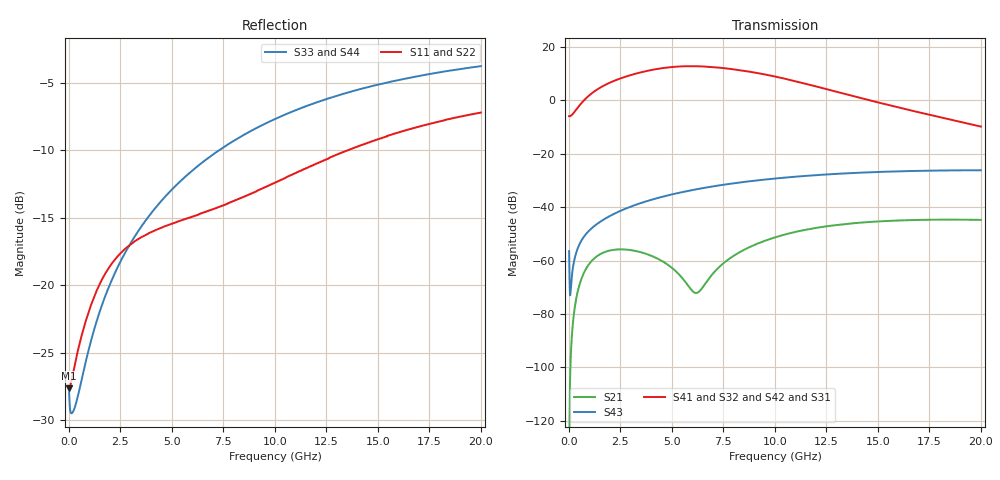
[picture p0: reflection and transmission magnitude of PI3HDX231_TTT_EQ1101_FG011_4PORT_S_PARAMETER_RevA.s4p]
! NPort=4 DATA=2000 NOISE=0 GROUPDELAY=0 COMPLEX_DATAFORMAT=POLAR
! NumOfBlock=1 NumOfParam=0
! .MODEL Smodel S TSTONEFILE=PI3HDX231_TTT_EQ1101_FG011_4PORT_S_PARAMETER_RevA.s4p TYPE=S
!  -- The above .MODEL line can be used for the S element in the netlist.
! The s parameter is extracted from the linear redriver, it is not bi-directional; only s(4,1)s(4,2) and s(3,1)s(3,2)
! should be the insertion loss
!Port definition:
!Port1 = input+
!Port2 = input-
!Port3 = output+
!Port4 = output-
# Hz S MA R  50
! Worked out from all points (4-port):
!   2000 points, 10 MHz to 20 GHz, reference 50 ohm
!   strongest paths, dB at 10 MHz, 5.01 GHz, 10.01 GHz, 15.01 GHz, 20 GHz:
!     S41: -5.9, 12.5, 8.9, -0.8, -9.9
!     S32: -5.9, 12.4, 8.8, -0.8, -9.8
!     S42: -5.9, 12.4, 8.8, -1.0, -10.0
!     S31: -5.9, 12.4, 8.7, -1.2, -10.2
!     S43: -56.5, -35.2, -29.3, -26.8, -26.2
!     S21: -134.8, -62.8, -51.3, -45.4, -44.8
!   lowest |S11| = -27.6 dB at 10 MHz (marker M1), VSWR 1.09, Z = 46 - j0.0776 ohm
!   |S11| at or under -10 dB: start of sweep to 13.55 GHz
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1e7  0.04152 -178.8  1.825e-07 -13.9  0 0.0  0 0.0
     1.825e-07 -14.0  0.04152 -178.8  0 0.0  0 0.0
     0.5043 0.4  0.5043 -179.6  0.04012 -3.2  0.0015 -70.3
     0.5043 -179.6  0.5043 0.4  0.0015 -70.3  0.04012 -3.2
3.38e9  0.1484 -140.9  0.001465 7.8  6.98e-11 -124.5  5.589e-11 -115.7
        0.001466 7.8  0.1485 -141.0  5.45e-11 -116.2  7.181e-11 -123.8
        3.222 -28.4  3.231 151.4  0.1593 -97.0  0.01153 69.4
        3.252 151.5  3.239 -27.8  0.01152 69.3  0.1594 -97.0
5.44e9  0.1736 -139.3  0.0004967 -8.4  1.184e-09 169.5  7.836e-10 -166.4
        0.0005006 -8.4  0.1736 -139.5  7.592e-10 -165.9  1.229e-09 169.3
        4.257 -93.6  4.276 86.2  0.2437 -103.8  0.01893 59.1
        4.309 86.1  4.294 -92.9  0.01887 59.0  0.2438 -103.8
7.58e9  0.1986 -134.5  0.0009462 102.7  7.926e-09 104.0  5.608e-09 138.5
        0.0009394 102.2  0.1981 -134.7  5.469e-09 139.9  8.211e-09 102.8
        3.904 -161.7  3.945 18.1  0.3264 -109.6  0.02657 46.2
        3.974 17.8  3.948 -160.8  0.02646 46.3  0.3265 -109.6
1.015e10  0.2424 -129.4  0.002835 83.7  3.538e-08 31.8  2.735e-08 65.2
          0.002818 83.4  0.2411 -129.6  2.706e-08 67.1  3.619e-08 30.0
          2.64 125.9  2.697 -54.5  0.4168 -116.0  0.03481 29.6
          2.709 -55.2  2.677 126.9  0.03469 29.7  0.4169 -116.0
1.33e10  0.3112 -128.3  0.004792 50.5  1.092e-07 -42.8  8.622e-08 -16.0
         0.004762 50.2  0.3092 -128.3  8.667e-08 -14.2  1.1e-07 -44.7
         1.293 55.0  1.345 -126.3  0.5104 -123.1  0.04257 8.9
         1.343 -127.0  1.318 56.2  0.04249 9.2  0.5103 -123.1
2e10  0.4356 -135.6  0.005806 -4.0  3.81e-07 -162.7  2.843e-07 -145.4
      0.005762 -4.2  0.4339 -135.4  2.898e-07 -144.5  3.781e-07 -164.1
      0.3078 -50.3  0.3254 124.7  0.6464 -135.0  0.04885 -32.3
      0.3217 124.2  0.317 -49.1  0.04895 -32.1  0.6461 -135.0
